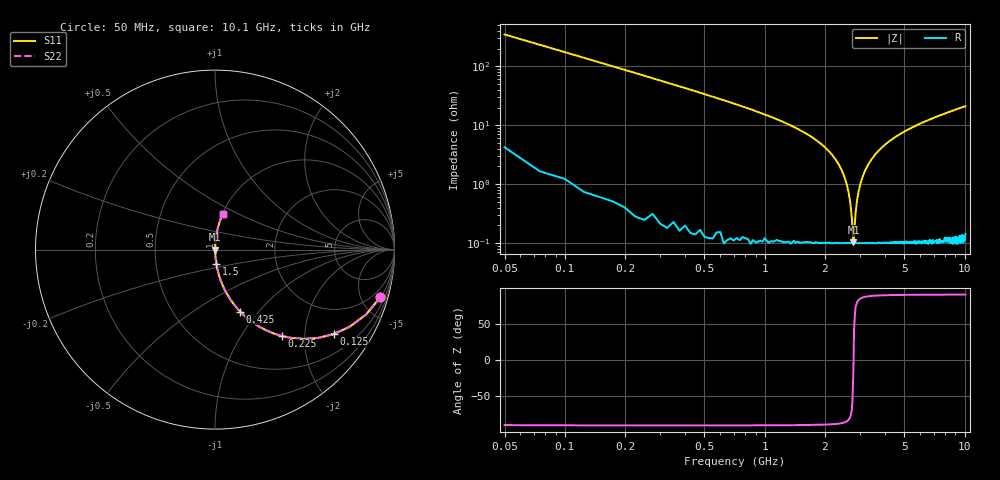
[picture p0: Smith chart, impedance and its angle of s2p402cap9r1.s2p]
! AVX Thin Film Operation		Date: April 2003
! Description: Accu-P® Series, Thin Film, SMD, RF Capacitor
! Part Number: 0402ZK9R1BBW
! 50 MHz  -  10.05 GHz
! Serial Measurements
# hz S db R 50
!	S11		S21		S12		S22
!	dB	Phase	dB	Phase	dB	Phase	dB	Phase
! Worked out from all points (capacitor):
!   400 points, 50 MHz to 10.1 GHz, reference 50 ohm
!   read as one part in series: C = 9.1 pF near 100 MHz
!   lowest |Z| = 103 mohm at 2.78 GHz (marker M1)
!   series resonance near 2.785 GHz, so ESL is about 360 pH
!   S11 on the Smith chart (normalised r, x): 50 MHz: 1.09, -7.00; 125 MHz: 1.02, -2.79; 225 MHz: 1.01, -1.54; 425 MHz: 1.00, -0.80; 1.5 GHz: 1.00, -0.17; 10.1 GHz: 1.00, +0.42
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5e7  -0.37 -15.9  -11.20 73.4  -11.20 73.4  -0.37 -15.9
7.5e7  -0.76 -23.2  -8.11 66.4  -8.11 66.4  -0.76 -23.2
1.25e8  -1.82 -35.5  -4.72 54.2  -4.72 54.2  -1.82 -35.5
2.25e8  -4.29 -52.2  -2.05 37.6  -2.05 37.6  -4.29 -52.2
4.25e8  -8.58 -67.9  -0.66 21.9  -0.66 21.9  -8.58 -67.9
8.25e8  -14.40 -78.7  -0.17 10.9  -0.17 10.9  -14.40 -78.7
1.5e9  -21.70 -84.6  -0.04 4.7  -0.04 4.7  -21.70 -84.6
1.73e9  -24.10 -85.5  -0.03 3.6  -0.03 3.6  -24.10 -85.5
2.18e9  -30.10 -86.4  -0.01 1.8  -0.01 1.8  -30.10 -86.4
2.53e9  -38.30 -84.6  -0.01 0.7  -0.01 0.7  -38.30 -84.6
2.68e9  -46.10 -78.1  -0.01 0.3  -0.01 0.3  -46.10 -78.1
2.73e9  -51.30 -68.4  -0.01 0.1  -0.01 0.1  -51.30 -68.4
2.78e9  -59.70 -14.4  -0.01 0.0  -0.01 0.0  -59.70 -14.4
2.85e9  -49.80 71.9  -0.01 -0.2  -0.01 -0.2  -49.80 71.9
2.95e9  -42.50 81.9  -0.01 -0.4  -0.01 -0.4  -42.50 81.9
3.15e9  -36.10 85.5  -0.01 -0.9  -0.01 -0.9  -36.10 85.5
3.4e9  -31.90 86.3  -0.01 -1.5  -0.01 -1.5  -31.90 86.3
4.15e9  -25.70 85.9  -0.02 -3.0  -0.02 -3.0  -25.70 85.9
5.08e9  -21.90 84.7  -0.04 -4.6  -0.04 -4.6  -21.90 84.7
6.75e9  -18.00 82.3  -0.08 -7.2  -0.08 -7.2  -18.00 82.3
8.43e9  -15.50 80.0  -0.13 -9.6  -0.13 -9.6  -15.50 80.0
1.01e10  -13.80 77.8  -0.20 -11.8  -0.20 -11.8  -13.80 77.8
